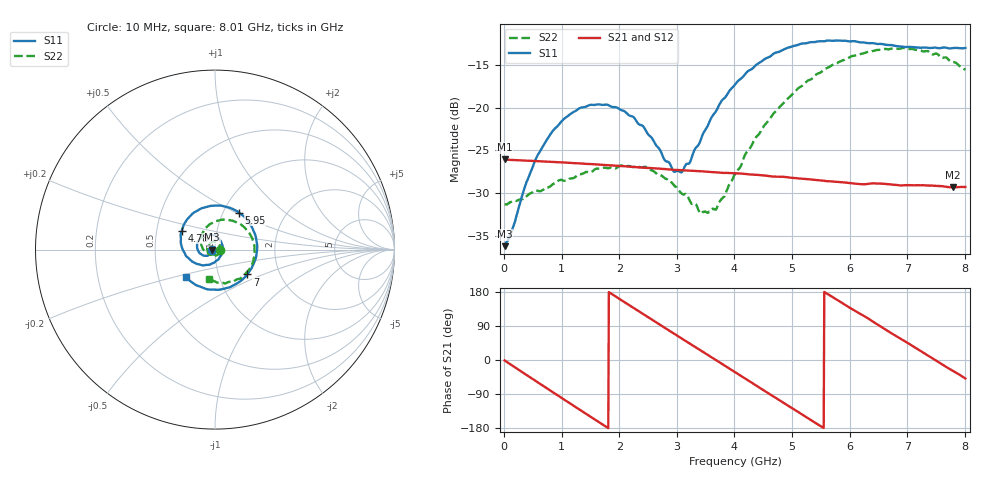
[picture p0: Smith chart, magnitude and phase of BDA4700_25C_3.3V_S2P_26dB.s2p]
!Agilent Technologies,E5071B,MY42404982,A.09.10
!Date: Mon Oct 20 18:14:00 2025
!Data & Calibration Information:
!Freq	S11:SOLT2(ON)	S21:SOLT2(ON)	S12:SOLT2(ON)	S22:SOLT2(ON)
# Hz S RI R 50
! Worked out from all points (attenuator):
!   801 points, 10 MHz to 8.01 GHz, reference 50 ohm
!   highest |S21| = -26.05 dB at 10 MHz (marker M1); lowest = -29.3 dB at 7.79 GHz (marker M2)
!   lowest |S11| = -36.2 dB at 10 MHz (marker M3), VSWR 1.03, Z = 48.5 - j0.113 ohm
!   |S11| at or under -10 dB: start of sweep to end of sweep
!   |S22| runs from -32.4 to -13.0 dB; largest |S21 - S12| = 0.00057
!   S11 on the Smith chart (normalised r, x): 10 MHz: 0.97, -0.00; 4.78 GHz: 0.67, +0.15; 5.95 GHz: 1.18, +0.52; 7 GHz: 1.37, -0.40; 8.01 GHz: 0.69, -0.22
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1e7  -0.0154 -0.00117  0.0498 -0.00105  0.0498 -0.00108  0.0271 -0.000834
1.3e8  -0.0164 -0.00925  0.0481 -0.0115  0.0481 -0.0114  0.0275 -0.0064
6e8  -0.0416 -0.0342  0.024 -0.0422  0.024 -0.0422  0.0131 -0.0297
1.01e9  -0.0806 -0.024  -0.00919 -0.0469  -0.00916 -0.0469  -0.0153 -0.0345
1.35e9  -0.0999 0.00921  -0.0331 -0.0335  -0.0331 -0.0335  -0.0366 -0.0182
2.08e9  -0.0476 0.0831  -0.0408 0.0201  -0.0408 0.0201  -0.0301 0.034
2.68e9  0.0313 0.0491  -0.00429 0.0438  -0.00436 0.0437  0.0131 0.0384
2.94e9  0.0416 0.00881  0.0144 0.0408  0.0144 0.0408  0.0256 0.0246
3.09e9  0.0385 -0.017  0.024 0.0357  0.0237 0.0358  0.0286 0.0126
3.41e9  0.00558 -0.0637  0.0383 0.0183  0.0383 0.0184  0.0213 -0.0113
3.55e9  -0.018 -0.0781  0.0412 0.00884  0.0412 0.00881  0.0131 -0.0205
3.7e9  -0.0484 -0.0851  0.0418 -0.00159  0.0418 -0.00169  0.000291 -0.0262
4.01e9  -0.1157 -0.0724  0.0351 -0.0219  0.0351 -0.0218  -0.0314 -0.0262
4.78e9  -0.1849 0.1058  -0.0109 -0.0379  -0.0106 -0.038  -0.0783 0.0629
5.35e9  -0.0659 0.2329  -0.0358 -0.0126  -0.0358 -0.0128  -0.0159 0.1473
5.95e9  0.1328 0.2066  -0.0291 0.022  -0.0291 0.0218  0.1191 0.152
6.37e9  0.2227 0.0866  -0.00916 0.0348  -0.00923 0.0346  0.1975 0.0805
6.68e9  0.2307 -0.0291  0.00922 0.0344  0.00932 0.0344  0.2198 -0.000251
7e9  0.1797 -0.1383  0.0245 0.0252  0.0246 0.025  0.2035 -0.0852
7.43e9  0.0389 -0.2207  0.0349 0.00312  0.0349 0.00307  0.1197 -0.1672
7.79e9  -0.0974 -0.2007  0.0301 -0.0161  0.03 -0.0161  0.0221 -0.1838
8.01e9  -0.1641 -0.1519  0.0226 -0.0258  0.0227 -0.0257  -0.0307 -0.1637
